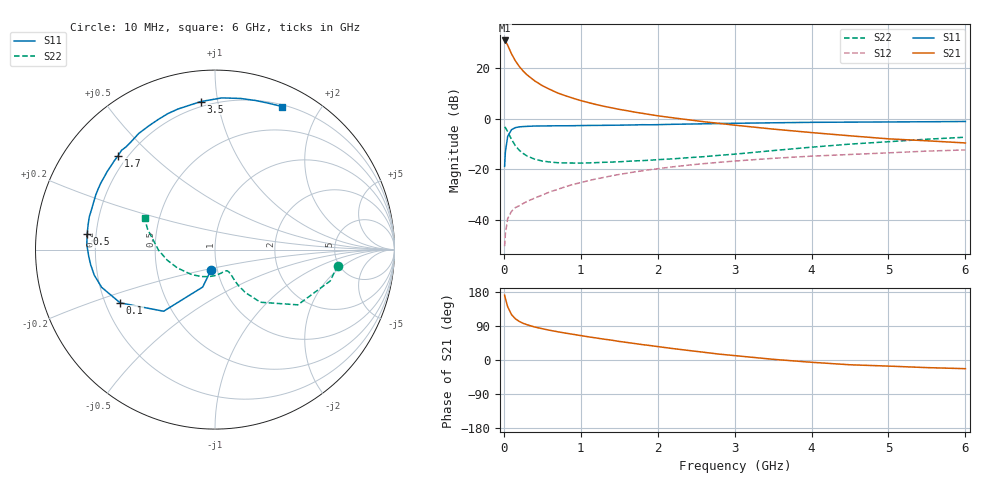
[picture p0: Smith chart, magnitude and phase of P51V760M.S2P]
! SIEMENS Small Signal Semiconductors
! BFP183
! Si NPN RF Bipolar Junction Transistor in SOT143
! VCE = 1.75 V  IC = 60 mA
! Common Emitter S-Parameters:  March  1996
# GHz  S  MA  R  50
!  f  S11  S21  S12  S22
! GHz  MAG  ANG  MAG  ANG  MAG  ANG  MAG  ANG
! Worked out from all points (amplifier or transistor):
!   36 points, 10 MHz to 6 GHz, reference 50 ohm
!   highest |S21| = 31.0 dB at 10 MHz (marker M1)
!   |S21| within 3 dB of that: start of sweep to 66.12 MHz
!   unconditionally stable (mu >= 1): start of sweep to 37.11 MHz; 155.5 MHz to end of sweep
!   at 250 MHz: K = 1.29, MAG = 23.0 dB, |S12| = -33.6 dB
!   at 1.4 GHz: K = 1.81, MAG = 8.2 dB, |S12| = -22.6 dB
!   at 6 GHz: K = 1.43, MAG = -2.5 dB, |S12| = -12.4 dB
!   S11 on the Smith chart (normalised r, x): 10 MHz: 0.94, -0.21; 100 MHz: 0.26, -0.24; 500 MHz: 0.17, +0.06; 1.7 GHz: 0.16, +0.40; 3.5 GHz: 0.17, +0.89; 6 GHz: 0.22, +1.55
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0.01  0.1141 -100.7  35.29 171.0  0.003 62.7  0.689 -7.4
0.02  0.2196 -108.2  34.41 162.3  0.0052 65.0  0.6654 -15.2
0.05  0.4471 -129.8  28.34 140.4  0.0106 56.4  0.5547 -33.7
0.1  0.606 -150.7  19.17 119.7  0.0147 45.8  0.3875 -49.2
0.15  0.6657 -161.6  13.94 108.7  0.0174 44.7  0.2918 -54.8
0.2  0.6877 -168.1  10.83 101.8  0.0189 46.2  0.2377 -57.0
0.25  0.6977 -173.0  8.807 96.9  0.0209 47.9  0.2055 -57.4
0.3  0.7043 -176.8  7.398 93.2  0.023 51.4  0.183 -57.4
0.4  0.7149 177.8  5.613 87.1  0.0268 54.5  0.158 -57.6
0.5  0.7174 173.1  4.498 82.6  0.0308 56.5  0.1451 -58.4
0.6  0.7203 169.0  3.783 78.3  0.0357 59.0  0.1386 -59.5
0.7  0.7238 165.4  3.225 74.5  0.0399 60.1  0.1345 -61.3
0.9  0.7258 158.9  2.538 67.8  0.05 61.3  0.1326 -66.1
1.1  0.7338 152.2  2.08 61.1  0.0594 61.0  0.1332 -71.8
1.3  0.7379 146.9  1.759 55.0  0.0688 60.1  0.137 -78.2
1.7  0.752 135.8  1.35 43.5  0.0884 57.2  0.146 -91.9
2.2  0.7741 123.3  1.039 30.1  0.1116 52.3  0.1604 -110.2
2.8  0.8019 109.1  0.807 15.5  0.1369 45.6  0.1882 -131.7
3.5  0.8285 95.5  0.622 1.8  0.1642 38.1  0.2336 -154.2
4.5  0.8542 80.3  0.458 -12.6  0.1956 27.2  0.3138 -179.2
5.5  0.8689 69.6  0.365 -20.1  0.2282 17.5  0.3922 163.2
6  0.8803 64.9  0.331 -22.9  0.2405 12.1  0.4295 156.0
